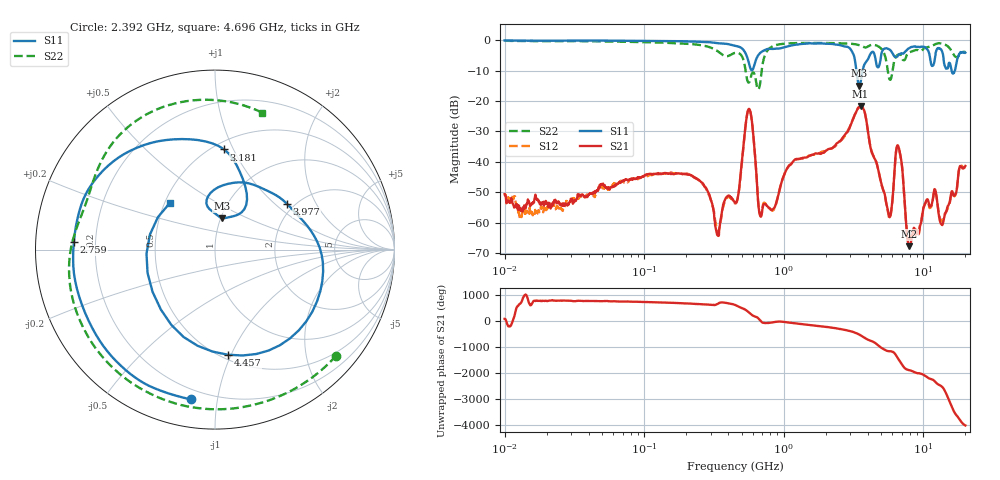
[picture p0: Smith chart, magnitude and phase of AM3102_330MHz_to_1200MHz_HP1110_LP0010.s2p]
! Date/Time: Tue, Sep 11, 2018 5:23 PM
! Network Analyzer: Agilent Technologies E8362B Rev: A.07.50.63
! Sweep from 0.010 to 20.000 GHz, 1601 Points, Sweep Type: LOG
! Power Supply: 4.949 V, 0.001 A
# Hz S DB R 50
!freq MagS11 AngS11 MagS21 AngS21 MagS12 AngS12 MagS22 AngS22
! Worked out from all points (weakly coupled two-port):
!   1601 points, 10 MHz to 20 GHz, reference 50 ohm
!   highest |S21| = -21.69 dB at 3.549 GHz (marker M1); lowest = -67.7 dB at 7.92 GHz (marker M2)
!   lowest |S11| = -15.0 dB at 3.482 GHz (marker M3), VSWR 1.44, Z = 50.6 + j18.2 ohm
!   |S11| at or under -10 dB: 3.312 GHz to 3.668 GHz (355.4 MHz wide, 10.2 % of centre); 15.92 GHz to 16.81 GHz (888.8 MHz wide, 5.43 % of centre)
!   |S22| runs from -16.1 to -0.2 dB; largest |S21 - S12| = 0.0052
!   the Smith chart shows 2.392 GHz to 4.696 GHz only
!   S11 on the Smith chart (normalised r, x): 2.392 GHz: 0.14, -0.84; 2.759 GHz: 0.12, +0.03; 3.181 GHz: 0.57, +0.92; 3.977 GHz: 1.83, +1.20; 4.457 GHz: 0.54, -0.97; 4.696 GHz: 0.53, +0.32
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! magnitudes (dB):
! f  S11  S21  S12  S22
! 10 MHz  0.0  -50.6  -50.7  -0.2
! 35.55 MHz  -0.1  -50.9  -51.3  -0.3
! 126.4 MHz  -0.2  -43.7  -44.0  -0.7
! 256.5 MHz  -0.5  -46.7  -46.8  -1.6
! 334.7 MHz  -0.9  -64.1  -62.9  -3.5
! 447.2 MHz  -1.8  -53.4  -53.7  -4.1
! 561.8 MHz  -7.4  -22.6  -22.6  -13.9
! 682.6 MHz  -4.0  -58.0  -57.6  -13.0
! 1.59 GHz  -1.0  -37.7  -37.7  -0.9
! 2.392 GHz  -1.5  -33.9  -34.4  -0.9
! 2.759 GHz  -2.1  -31.0  -31.3  -1.0
! 3.181 GHz  -5.0  -25.1  -25.1  -1.2
! 3.482 GHz  -15.0  -22.0  -21.9  -1.6
! 3.549 GHz  -13.8  -21.7  -21.6  -1.7
! 3.977 GHz  -6.5  -29.0  -28.8  -2.1
! 4.457 GHz  -4.6  -38.8  -38.7  -1.5
! 4.696 GHz  -8.8  -41.6  -41.7  -1.9
! 5.652 GHz  -2.9  -57.4  -57.9  -12.1
! 6.643 GHz  -4.7  -35.1  -35.2  -4.7
! 7.92 GHz  -2.5  -67.7  -65.5  -4.0
! 13.68 GHz  -3.9  -60.8  -59.4  -1.1
! 20 GHz  -4.1  -41.4  -41.9  -3.8
